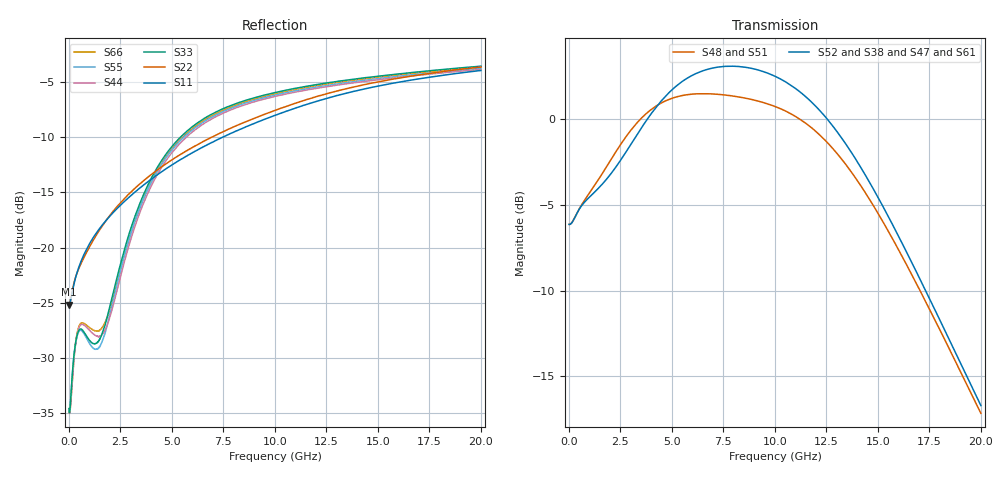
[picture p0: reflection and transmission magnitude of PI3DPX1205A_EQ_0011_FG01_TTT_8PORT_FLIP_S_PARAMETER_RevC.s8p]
! NPort=8 DATA=2000 NOISE=0 GROUPDELAY=0 COMPLEX_DATAFORMAT=POLAR
! NumOfBlock=1 NumOfParam=0
! .MODEL Smodel S TSTONEFILE=PI3DPX1205A_EQ_0011_FG01_TTT_8PORT_FLIP_S_PARAMETER_RevC.s8p TYPE=S
!  -- The above .MODEL line can be used for the S element in the netlist.
! The s parameter is extracted from the linear redriver, it is not bi-directional;
! only s(5,1)s(6,2)s(3,7)s(4,8) should be the insertion loss
!  Port definition:
!  Port1 = AIP
!  Port2 = AIN
!  Port3 = BOP
!  Port4 = BON
!  Port5 = AOP
!  Port6 = AON
!  Port7 = BIP
!  Port8 = BIN
# Hz S MA R  50
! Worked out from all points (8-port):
!   2000 points, 10 MHz to 20 GHz, reference 50 ohm
!   strongest paths, dB at 10 MHz, 5.01 GHz, 10.01 GHz, 15.01 GHz, 20 GHz:
!     S52: -6.1, 1.7, 2.5, -4.6, -16.7
!     S38: -6.1, 1.7, 2.5, -4.6, -16.7
!     S47: -6.1, 1.7, 2.5, -4.6, -16.6
!     S61: -6.1, 1.7, 2.5, -4.6, -16.6
!     S48: -6.1, 1.2, 0.7, -5.5, -17.2
!     S51: -6.1, 1.2, 0.7, -5.5, -17.2
!   lowest |S11| = -25.2 dB at 10 MHz (marker M1), VSWR 1.12, Z = 44.8 - j0.115 ohm
!   |S11| at or under -10 dB: start of sweep to 7.469 GHz
